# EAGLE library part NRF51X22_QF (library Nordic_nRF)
nRF51x22 For devices: nRF51422 nRF51822 Features Single chip, highly flexible, 2.4 GHz multi-protocol device 32-bit ARM Cortex M0 CPU core 256kB/128kB flash + 32kB/16kB RAM Supports Bluetooth low energy protocol stacks Thread safe and run-time protected Event driven API On air compatible with nRF24L series 3 data rates (2Mbps/1Mbps/250kbps) +4dBm output power -93dBm sensitivity, Bluetooth low energy PPI system for maximum power-efficient applications and code simplification Flexible power management system with automatic power management of each peripheral Configurable I/O mapping for analog and digital I/O Applications Mobile phone accessories Wearables Beacons Rezence wireless charging monitoring PC peripherals Consumer Electronics (CE) remote controls Proximity/Alert sensors Smart Home Sports, fitness and healthcare sensors Smart RF tags Toys and electronic games Intelligent domestic appliances Industrial and commercial sensors Lighting
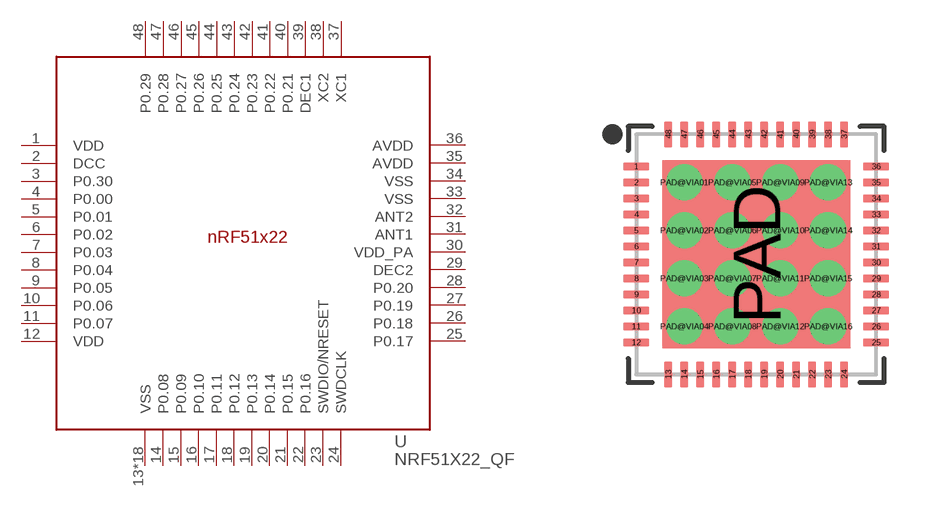
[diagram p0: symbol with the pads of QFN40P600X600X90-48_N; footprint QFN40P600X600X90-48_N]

Designator prefix -

## NRF51X22_QFQF  [QFN40P600X600X90-48_N]
1  VDD  pwr
2  DCC  pwr
3  P0.30
4  P0.00
5  P0.01
6  P0.02
7  P0.03
8  P0.04
9  P0.05
10  P0.06
11  P0.07
12  VDD  pwr
13  VSS  pwr
14  P0.08
15  P0.09
16  P0.10
17  P0.11
18  P0.12
19  P0.13
20  P0.14
21  P0.15
22  P0.16
23  SWDIO/NRESET
24  SWDCLK  in
25  P0.17
26  P0.18
27  P0.19
28  P0.20
29  DEC2  pwr
30  VDD_PA  pwr
31  ANT1
32  ANT2
33  VSS  pwr
34  VSS  pwr
35  AVDD  pwr
36  AVDD  pwr
37  XC1
38  XC2
39  DEC1  pwr
40  P0.21
41  P0.22
42  P0.23
43  P0.24
44  P0.25
45  P0.26
46  P0.27
47  P0.28
48  P0.29
PAD  VSS  pwr
PAD@VIA01  VSS  pwr
PAD@VIA02  VSS  pwr
PAD@VIA03  VSS  pwr
PAD@VIA04  VSS  pwr
PAD@VIA05  VSS  pwr
PAD@VIA06  VSS  pwr
PAD@VIA07  VSS  pwr
PAD@VIA08  VSS  pwr
PAD@VIA09  VSS  pwr
PAD@VIA10  VSS  pwr
PAD@VIA11  VSS  pwr
PAD@VIA12  VSS  pwr
PAD@VIA13  VSS  pwr
PAD@VIA14  VSS  pwr
PAD@VIA15  VSS  pwr
PAD@VIA16  VSS  pwr

## Footprint QFN40P600X600X90-48_N (pad centres in mm)
QFN40P600X600X90-48N QFN, 48-Leads Body 6.0x6.0mm (max) Pitch 0.40mm IPC Medium Density
smd 0.65 x 0.2: 1 -3,2.2; 2 -3,1.8; 3 -3,1.4; 4 -3,1; 5 -3,0.6; 6 -3,0.2; 7 -3,-0.2; 8 -3,-0.6; 9 -3,-1; 10 -3,-1.4; 11 -3,-1.8; 12 -3,-2.2; 25 3,-2.2; 26 3,-1.8; 27 3,-1.4; 28 3,-1; 29 3,-0.6; 30 3,-0.2; 31 3,0.2; 32 3,0.6; 33 3,1; 34 3,1.4; 35 3,1.8; 36 3,2.2
smd 0.2 x 0.65: 13 -2.2,-3; 14 -1.8,-3; 15 -1.4,-3; 16 -1,-3; 17 -0.6,-3; 18 -0.2,-3; 19 0.2,-3; 20 0.6,-3; 21 1,-3; 22 1.4,-3; 23 1.8,-3; 24 2.2,-3; 37 2.2,3; 38 1.8,3; 39 1.4,3; 40 1,3; 41 0.6,3; 42 0.2,3; 43 -0.2,3; 44 -0.6,3; 45 -1,3; 46 -1.4,3; 47 -1.8,3; 48 -2.2,3
smd 4.7 x 4.7: PAD 0,0
drill 0.4: PAD@VIA01 -1.8,1.8; PAD@VIA02 -1.8,0.6; PAD@VIA03 -1.8,-0.6; PAD@VIA04 -1.8,-1.8; PAD@VIA05 -0.6,1.8; PAD@VIA06 -0.6,0.6; PAD@VIA07 -0.6,-0.6; PAD@VIA08 -0.6,-1.8; PAD@VIA09 0.6,1.8; PAD@VIA10 0.6,0.6; PAD@VIA11 0.6,-0.6; PAD@VIA12 0.6,-1.8; PAD@VIA13 1.8,1.8; PAD@VIA14 1.8,0.6; PAD@VIA15 1.8,-0.6; PAD@VIA16 1.8,-1.8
